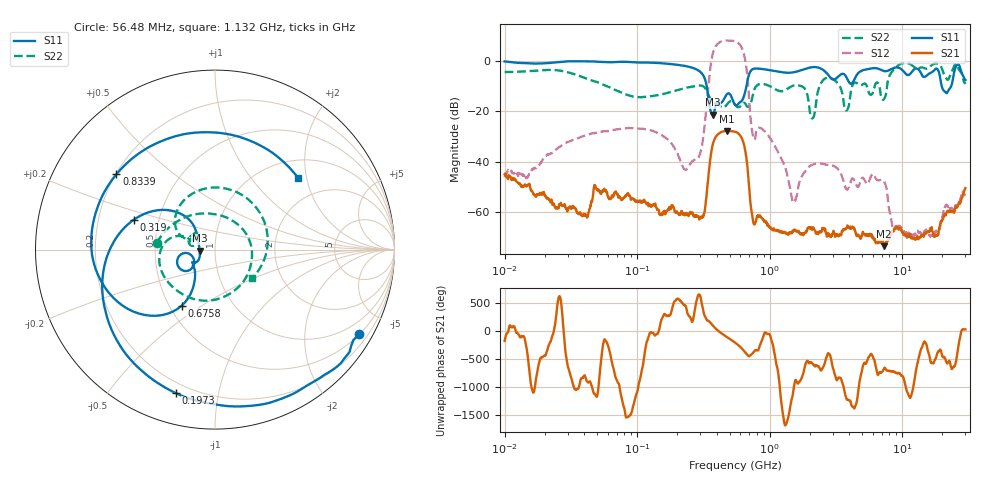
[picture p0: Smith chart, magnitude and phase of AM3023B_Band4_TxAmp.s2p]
# Hz S DB R 50.0
!freq dBS11 angS11 dBS21 angS21 dBS12 angS12 dBS22 angS22
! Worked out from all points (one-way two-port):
!   1601 points, 10 MHz to 30 GHz, reference 50 ohm
!   highest |S21| = -27.76 dB at 473.7 MHz (marker M1); lowest = -73.3 dB at 7.316 GHz (marker M2)
!   lowest |S11| = -21.4 dB at 370.7 MHz (marker M3), VSWR 1.19, Z = 42.1 - j0.501 ohm
!   |S11| at or under -10 dB: 334.7 MHz to 668.8 MHz (334.1 MHz wide, 66.6 % of centre); 19.86 GHz to 23.47 GHz (3.617 GHz wide, 16.7 % of centre)
!   |S22| runs from -22.9 to -0.9 dB; largest |S21 - S12| = 2.5
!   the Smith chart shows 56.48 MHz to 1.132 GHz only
!   S11 on the Smith chart (normalised r, x): 56.48 MHz: 0.51, -3.63; 197.3 MHz: 0.15, -0.75; 319 MHz: 0.36, +0.16; 675.8 MHz: 0.58, -0.42; 833.9 MHz: 0.20, +0.33; 1.132 GHz: 1.41, +1.79
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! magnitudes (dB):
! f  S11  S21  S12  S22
! 10 MHz  -0.3  -44.9  -46.1  -4.5
! 38.04 MHz  -0.3  -61.1  -30.1  -6.4
! 56.48 MHz  -0.6  -50.6  -27.9  -9.7
! 144.7 MHz  -1.0  -58.9  -28.8  -13.6
! 197.3 MHz  -1.6  -60.2  -35.9  -11.8
! 236.3 MHz  -2.3  -60.2  -43.0  -10.7
! 319 MHz  -6.3  -60.6  -28.3  -10.4
! 370.7 MHz  -21.4  -33.5  2.3  -16.5
! 473.7 MHz  -13.4  -27.8  7.9  -17.5
! 547.7 MHz  -17.5  -28.1  7.6  -17.4
! 675.8 MHz  -8.8  -40.7  -5.1  -18.2
! 747 MHz  -3.4  -63.1  -29.6  -13.6
! 833.9 MHz  -3.2  -61.4  -26.6  -9.3
! 1.132 GHz  -4.3  -67.3  -35.1  -11.6
! 1.52 GHz  -4.6  -67.2  -56.1  -9.9
! 2.084 GHz  -2.6  -66.8  -41.2  -22.8
! 2.703 GHz  -5.0  -69.5  -41.2  -6.8
! 3.798 GHz  -6.6  -66.1  -50.8  -19.7
! 7.316 GHz  -4.2  -73.3  -47.8  -15.2
! 7.926 GHz  -3.9  -70.4  -58.0  -6.7
! 16.54 GHz  -4.8  -66.2  -69.3  -2.0
! 30 GHz  -7.7  -50.3  -53.0  -9.3
